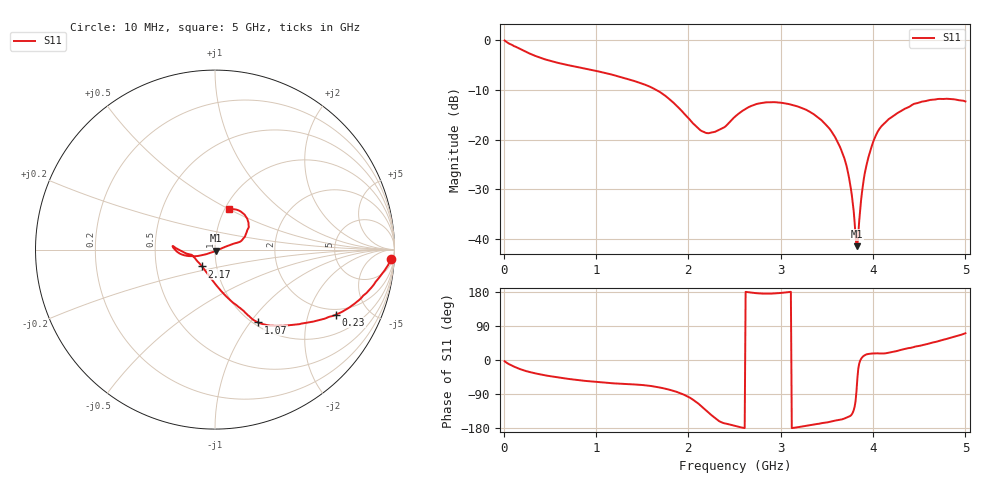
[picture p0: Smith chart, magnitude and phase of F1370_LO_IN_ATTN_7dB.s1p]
! S-parameters for LO input IDT F1370 DPD Demodulator
! Date Measured:  2015-11-25  RGG
!  Port 1 = Pin 12 = LO_IN
! State: 7 dB attenuation (Gain = Gmax - 7 dB)
! LO Frequency:  10 MHz to 5000 MHz
! RF_INX, RF_INY, IF_I+, IF_I-, IF_Q+, and IF_Q- terminated
! Vcc = +5.00 Volts  Icc = approx 275 mA.
! NOTES:  The device was measured on a custom printed circuit evaluation board with individual 50 ohm
!  microstrip lines to the RF and LO pins. The 50 ohm microstrip lines were de-embedded using reference
!  plane extensions
! Frequency Re{S11} Im{S11}
# HZ  S  RI R 50.00
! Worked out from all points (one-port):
!   500 points, 10 MHz to 5 GHz, reference 50 ohm
!   lowest |S11| = -41.4 dB at 3.83 GHz (marker M1), VSWR 1.02, Z = 50.6 - j0.655 ohm
!   |S11| at or under -10 dB: 1.647 GHz to end of sweep
!   S11 on the Smith chart (normalised r, x): 10 MHz: 11, -34; 230 MHz: 1.74, -3.05; 1.07 GHz: 1.05, -1.09; 2.17 GHz: 0.85, -0.16; 5 GHz: 1.05, +0.51
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1e7  0.9822 -0.0523
1.1e8  0.8253 -0.2568
2.3e8  0.6738 -0.3624
4e8  0.5174 -0.4063
6.4e8  0.3834 -0.4242
1.07e9  0.24 -0.4062
1.26e9  0.196 -0.3766
1.65e9  0.1029 -0.2978
1.89e9  0.0161 -0.2096
2.17e9  -0.0735 -0.0936
2.37e9  -0.1257 -0.0327
2.51e9  -0.1703 -0.0168
2.76e9  -0.2292 0.0162
3.13e9  -0.2213 -0.00239
3.35e9  -0.179 -0.0296
3.55e9  -0.1146 -0.0373
3.68e9  -0.0624 -0.0285
3.76e9  -0.0268 -0.0178
3.81e9  -0.00373 -0.0105
3.83e9  0.00557 -0.00648
3.84e9  0.0102 -0.0044
3.88e9  0.0294 0.00324
3.91e9  0.0447 0.00996
4.01e9  0.095 0.0299
4.14e9  0.1433 0.0461
4.38e9  0.18 0.1089
4.7e9  0.1663 0.193
5e9  0.0803 0.2273
